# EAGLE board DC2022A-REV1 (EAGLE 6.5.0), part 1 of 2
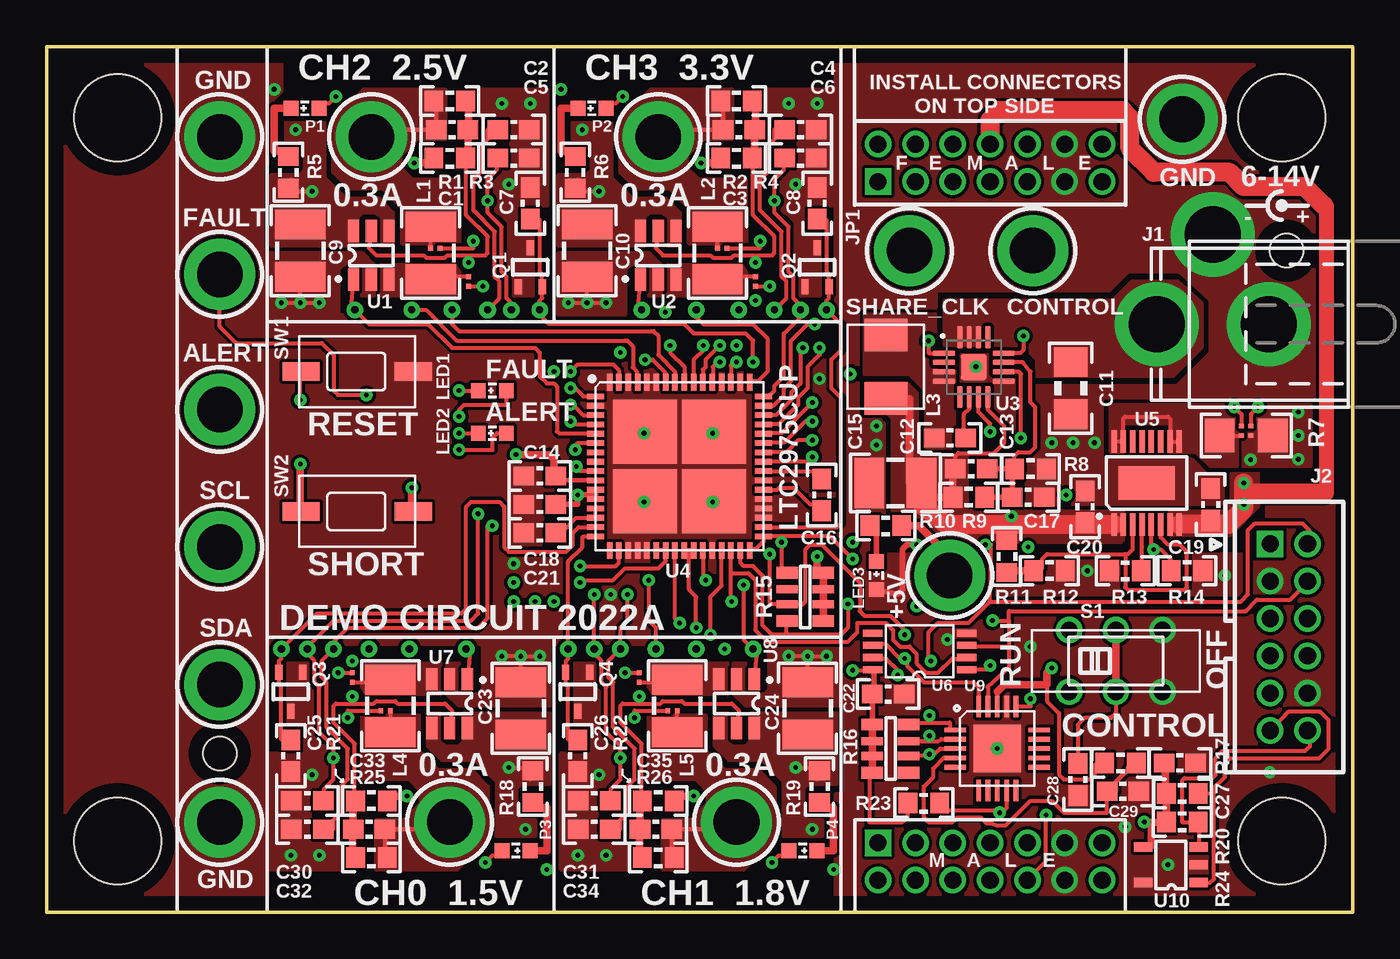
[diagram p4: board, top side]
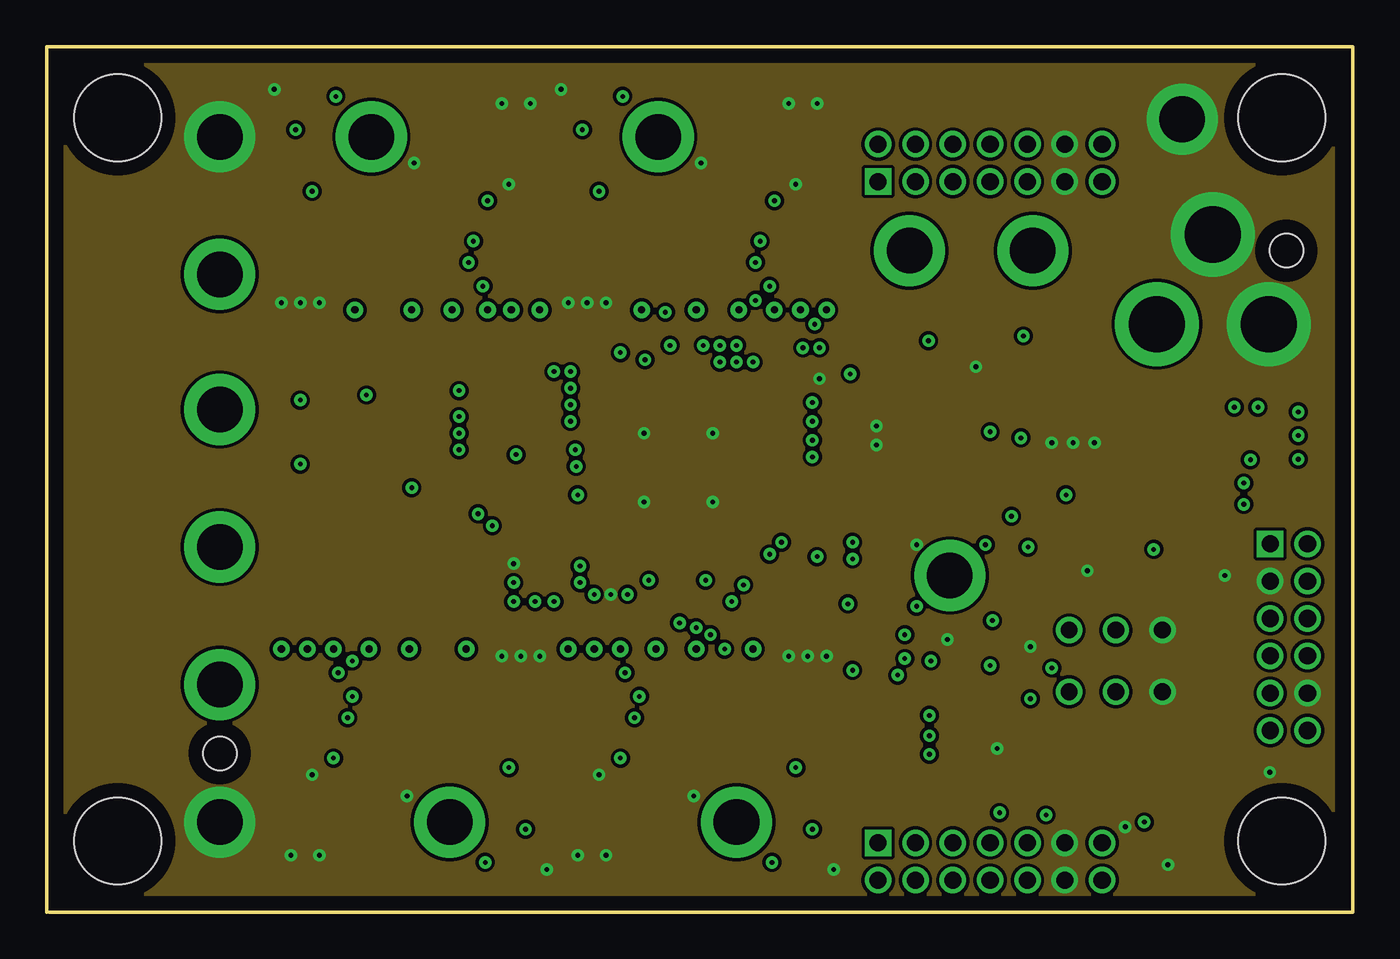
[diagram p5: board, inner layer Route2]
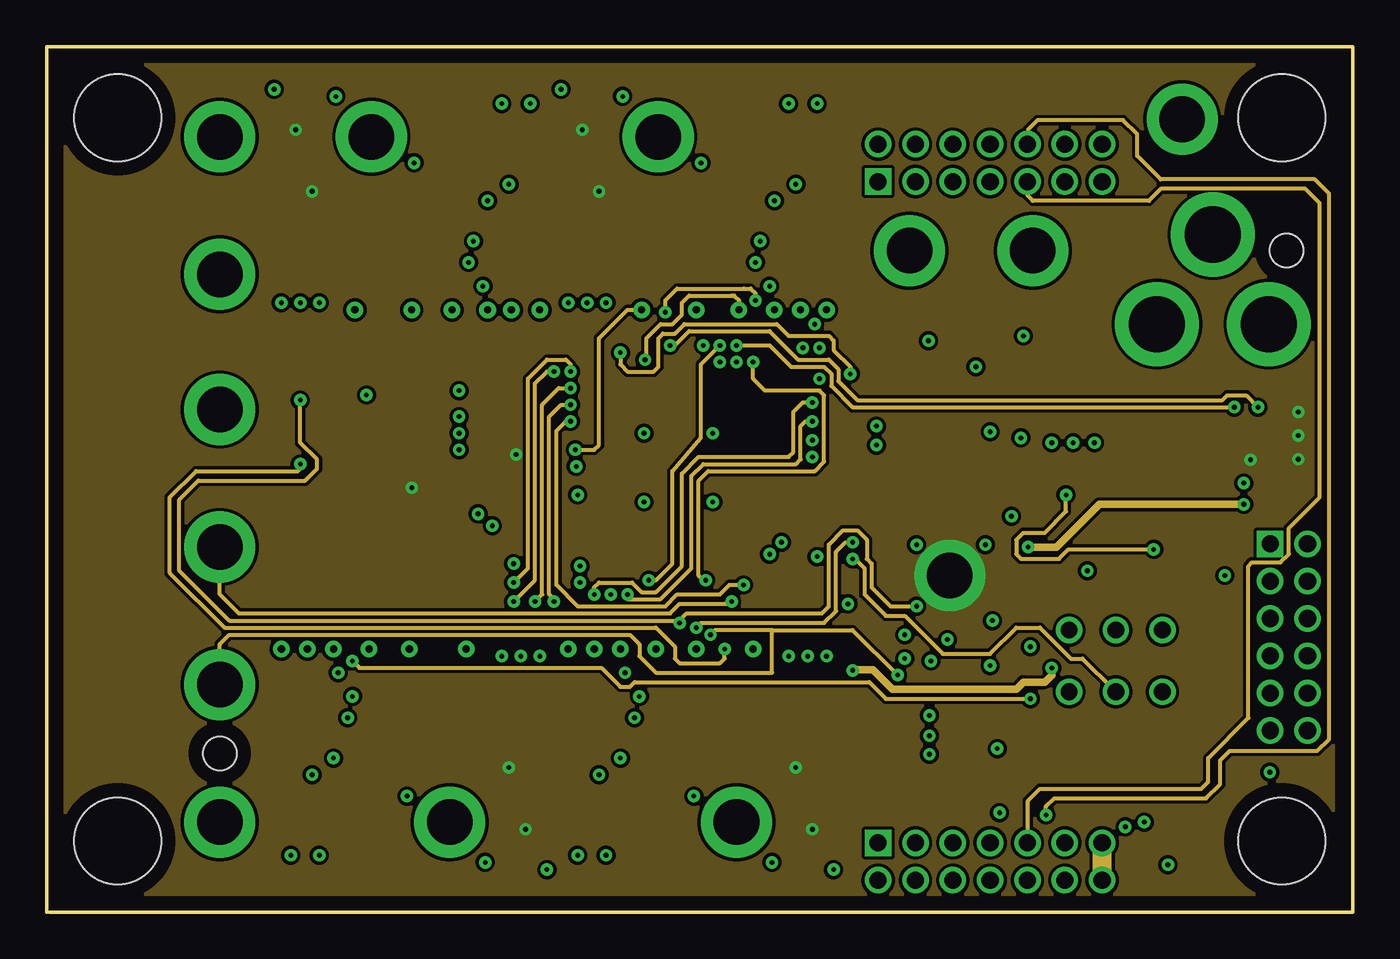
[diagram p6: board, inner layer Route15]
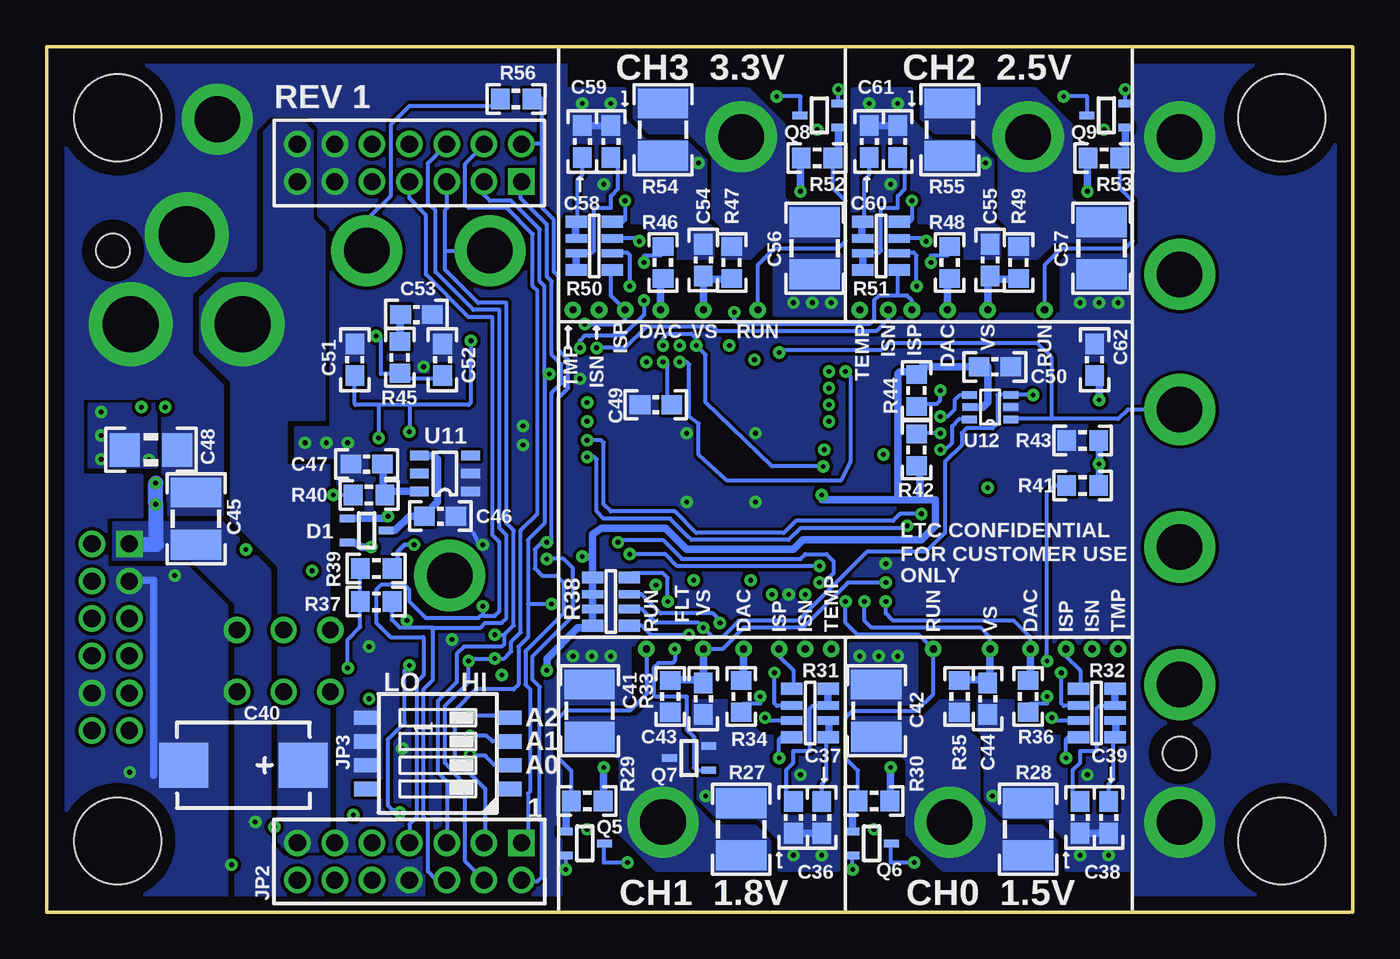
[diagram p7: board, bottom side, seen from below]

Size 69.98 x 46.35 mm. Coordinates in mm from the lower left corner, seen from the top.
Outline: 0,0 0,46.35 69.98,46.35 69.98,0 0.13,0
Copper layers (1*2+15*16): Top 0.035mm / dielectric 1.5mm / Route2 0.035mm / dielectric 0.15mm / Route15 0.035mm / dielectric 0.2mm / Bottom 0.035mm
Design rules "default *": minimum track width 8mil, minimum drill 10mil, track to track 7mil, track to pad 7mil, pad to pad 7mil, via to via 7mil, smd to smd 4mil, copper to edge 30mil, drill to drill 15mil, minimum pad ring 10mil, minimum via ring 8mil, stop-mask expansion 4mil, vias tented up to drill 16mil, thermal gap 10mil
Holes 4.65 mm at 3.81,3.81 3.81,42.55 66.17,42.55 66.17,3.81
Holes 1.8 mm at 66.42,35.43 9.27,8.51

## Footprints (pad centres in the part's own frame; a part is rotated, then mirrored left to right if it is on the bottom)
C0603_BOX = smd 1.1 x 1: 1 -0.85,0; 2 0.85,0
C1210_BOX = smd 1.6 x 2.7: 1 -1.4,0; 2 1.4,0
C1206_BOX = smd 1.6 x 1.8: 1 -1.4,0; 2 1.4,0
C7343 = smd 2.6 x 2.4: + -3.2,0; - 3.2,0
SC70-3 = smd 0.4 x 0.8: 1 -0.65,-1.052; 2 0.65,-1.052; 3 0,1.052
PJ-002A = drill 3 pad 4.5: 1 -3,0; 2 0,-4.8; 3 3,0
CONN_DC1613 = drill 0.914 square: 1 -5,-1 | drill 0.914: 2 -5,1; 3 -3,-1; 4 -3,1; 5 -1,-1; 6 -1,1; 7 1,-1; 8 1,1; 9 3,-1; 10 3,1; 11 5,-1; 12 5,1
2X07M = drill 0.914 square: 1 -6,-1 | drill 0.914: 2 -6,1; 3 -4,-1; 4 -4,1; 5 -2,-1; 6 -2,1; 7 0,-1; 8 0,1; 9 2,-1; 10 2,1; 11 4,-1; 12 4,1; 13 6,-1; 14 6,1
SMT_DIP_4 = smd 1.27 x 0.762: 1 -3.861,1.905; 2 -3.861,0.635; 3 -3.861,-0.635; 4 -3.861,-1.905; 5 3.861,-1.905; 6 3.861,-0.635; 7 3.861,0.635; 8 3.861,1.905
L1210 = smd 1.6 x 2.7: 1 -1.4,0; 2 1.4,0
IHLP_1616AB = smd 1.75 x 2.3: 1 -1.7,0; 2 1.7,0
CHIPLED_0603 = smd 0.8 x 0.8: N 0,0.75; P 0,-0.75
NODE_BREAKER = smd 0.254 x 0.254: 1 -0.254,0; 2 0.254,0
R0603_BOX = smd 1 x 1.1: 1 -0.85,0; 2 0.85,0
R1206_BOX = smd 1.6 x 1.803: 1 -1.422,0; 2 1.422,0
R_VISHAY_CRA06S = smd 1.15 x 0.63: R1_1 -0.975,1.295; R1_2 0.975,1.295; R4_1 -0.975,-1.295; R4_2 0.975,-1.295 | smd 1.15 x 0.44: R2_1 -0.975,0.4; R2_2 0.975,0.4; R3_1 -0.975,-0.4; R3_2 0.975,-0.4
R1210_BOX = smd 1.6 x 2.7: 1 -1.4,0; 2 1.4,0
JS202011CQN = drill 0.9: 1 -2.5,1.65; 2 0,1.65; 3 2.5,1.65; 4 -2.5,-1.65; 5 0,-1.65; 6 2.5,-1.65
SWITCH_PTS635 = smd 2 x 1: SW1 -3,0; SW2 3,0
TP1 = drill 2.438 pad 3.81: TP 0,0
VIA = drill 0.381: 1 0,0
SOT-23-6 = smd 1.2 x 0.6: 1 -1.3,0.95; 2 -1.3,0; 3 -1.3,-0.95; 4 1.3,-0.95; 5 1.3,0; 6 1.3,0.95
QFN16_3X3 = smd 1.2 x 0.3: 1 -1.711,0.734; 2 -1.711,0.234; 3 -1.711,-0.266; 4 -1.711,-0.766; 9 1.489,-0.766; 10 1.489,-0.266; 11 1.489,0.234; 12 1.489,0.734 | smd 0.3 x 1.2: 5 -0.861,-1.616; 6 -0.361,-1.616; 7 0.139,-1.616; 8 0.639,-1.616; 13 0.639,1.584; 14 0.139,1.584; 15 -0.361,1.584; 16 -0.861,1.584 | smd 1.4 x 1.4: PAD -0.111,-0.016
QFN64_9X9 = smd 0.9 x 0.3: 1 -4.5,3.75; 2 -4.5,3.25; 3 -4.5,2.75; 4 -4.5,2.25; 5 -4.5,1.75; 6 -4.5,1.25; 7 -4.5,0.75; 8 -4.5,0.25; 9 -4.5,-0.25; 10 -4.5,-0.75; 11 -4.5,-1.25; 12 -4.5,-1.75; 13 -4.5,-2.25; 14 -4.5,-2.75; 15 -4.5,-3.25; 16 -4.5,-3.75; 33 4.5,-3.75; 34 4.5,-3.25; 35 4.5,-2.75; 36 4.5,-2.25; 37 4.5,-1.75; 38 4.5,-1.25; 39 4.5,-0.75; 40 4.5,-0.25; 41 4.5,0.25; 42 4.5,0.75; 43 4.5,1.25; 44 4.5,1.75; 45 4.5,2.25; 46 4.5,2.75; 47 4.5,3.25; 48 4.5,3.75 | smd 0.3 x 0.9: 17 -3.75,-4.5; 18 -3.25,-4.5; 19 -2.75,-4.5; 20 -2.25,-4.5; 21 -1.75,-4.5; 22 -1.25,-4.5; 23 -0.75,-4.5; 24 -0.25,-4.5; 25 0.25,-4.5; 26 0.75,-4.5; 27 1.25,-4.5; 28 1.75,-4.5; 29 2.25,-4.5; 30 2.75,-4.5; 31 3.25,-4.5; 32 3.75,-4.5; 49 3.75,4.5; 50 3.25,4.5; 51 2.75,4.5; 52 2.25,4.5; 53 1.75,4.5; 54 1.25,4.5; 55 0.75,4.5; 56 0.25,4.5; 57 -0.25,4.5; 58 -0.75,4.5; 59 -1.25,4.5; 60 -1.75,4.5; 61 -2.25,4.5; 62 -2.75,4.5; 63 -3.25,4.5; 64 -3.75,4.5 | smd 3.429 x 3.429: PAD1 -1.854,1.854; PAD2 1.854,1.854; PAD3 -1.854,-1.854; PAD4 1.854,-1.854
MSOP16_EXP = smd 1.2 x 0.3: 1 -2.213,1.75; 2 -2.213,1.25; 3 -2.213,0.75; 4 -2.213,0.25; 5 -2.213,-0.25; 6 -2.213,-0.75; 7 -2.213,-1.25; 8 -2.213,-1.75; 9 2.213,-1.75; 10 2.213,-1.25; 11 2.213,-0.75; 12 2.213,-0.25; 13 2.213,0.25; 14 2.213,0.75; 15 2.213,1.25; 16 2.213,1.75 | smd 1.778 x 3.048: EXP 0,0
MSOP-8 = smd 1.041 x 0.381: 1 -2.55,0.975; 2 -2.55,0.325; 3 -2.55,-0.325; 4 -2.55,-0.975; 5 2.479,-0.975; 6 2.479,-0.325; 7 2.479,0.325; 8 2.479,0.975
QFN20 = smd 1.143 x 0.254: 1 -2.25,1; 2 -2.25,0.5; 3 -2.25,0; 4 -2.25,-0.5; 5 -2.25,-1; 11 2.25,-1; 12 2.25,-0.5; 13 2.25,0; 14 2.25,0.5; 15 2.25,1 | smd 0.254 x 1.143: 6 -1,-2.25; 7 -0.5,-2.25; 8 0,-2.25; 9 0.5,-2.25; 10 1,-2.25; 16 1,2.25; 17 0.5,2.25; 18 0,2.25; 19 -0.5,2.25; 20 -1,2.25 | smd 2.54 x 2.54: PAD 0,0
SOT-23-5 = smd 1 x 0.5: 1 -1.649,0.95; 2 -1.649,0; 3 -1.649,-0.95; 4 1.333,-0.95; 5 1.333,0.95
SOT-23-6@1 = smd 1 x 0.5: 1 -1.374,1.087; 2 -1.374,0.127; 3 -1.374,-0.833; 4 1.374,-0.833; 5 1.374,0.127; 6 1.374,1.087
SC70-6 = smd 0.4 x 0.8: 1 -0.65,-1.102; 2 0,-1.102; 3 0.65,-1.102; 4 0.65,1.102; 5 0,1.098; 6 -0.65,1.102

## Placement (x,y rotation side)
$$U$1  [LT_LOGO_LARGE_SM]  5.46,6.1 90 top
$$U$2  [LT_LOGO_LARGE_SM]  2.03,6.1 90 bottom
C1  220p  [C0603_BOX]  21.72,41.91 0 top
C2  2.2n  [C0603_BOX]  25.02,41.91 0 top
C3  220p  [C0603_BOX]  37.08,41.91 0 top
C4  2.2n  [C0603_BOX]  40.39,41.91 0 top
C5  2.2n  [C0603_BOX]  25.02,40.39 0 top
C6  2.2n  [C0603_BOX]  40.39,40.39 0 top
C7  100n  [C0603_BOX]  25.91,37.97 90 top
C8  100n  [C0603_BOX]  41.27,37.97 90 top
C9  22u/10V  [C1210_BOX]  13.59,35.43 270 top
C10  22u/10V  [C1210_BOX]  28.96,35.43 270 top
C11  10u/25V  [C1206_BOX]  54.86,28.07 90 top
C12  100n  [C0603_BOX]  48.39,25.4 0 top
C13  68p  [C0603_BOX]  49.53,23.75 0 top
C14  1u  [C0603_BOX]  26.42,23.37 0 top
C15  22u/10V  [C1210_BOX]  45.47,22.99 180 top
C16  100n  [C0603_BOX]  41.53,22.35 270 top
C17  47p  [C0603_BOX]  52.58,22.23 0 top
C18  100n  [C0603_BOX]  26.42,21.84 0 top
C19  1u  [C0603_BOX]  62.36,21.84 90 top
C20  1u  [C0603_BOX]  55.63,21.72 90 top
C21  100n  [C0603_BOX]  26.42,20.32 0 top
C22  100n  [C0603_BOX]  45.09,11.68 0 top
C23  22u/10V  [C1210_BOX]  25.4,10.92 90 top
C24  22u/10V  [C1210_BOX]  40.77,10.92 90 top
C25  100n  [C0603_BOX]  13.08,8.38 270 top
C26  100n  [C0603_BOX]  28.45,8.38 270 top
C27  1u  [C0603_BOX]  60.71,8 0 top
C28  1u  [C0603_BOX]  55.24,7.11 270 top
C29  1u  [C0603_BOX]  57.66,6.48 0 top
C30  2.2n  [C0603_BOX]  13.97,5.97 180 top
C31  2.2n  [C0603_BOX]  29.34,5.97 180 top
C32  2.2n  [C0603_BOX]  13.97,4.45 180 top
C33  220p  [C0603_BOX]  17.27,4.45 180 top
C34  2.2n  [C0603_BOX]  29.34,4.45 180 top
C35  220p  [C0603_BOX]  32.64,4.45 180 top
C36  10n  [C0603_BOX]  29.97,5.08 90 bottom
C37  10n  [C0603_BOX]  28.45,5.08 270 bottom
C38  10n  [C0603_BOX]  14.61,5.08 90 bottom
C39  10n  [C0603_BOX]  13.08,5.08 270 bottom
C40  47u/16V  [C7343]  59.44,7.87 180 bottom
C41  22u/10V  [C1210_BOX]  40.89,10.79 90 bottom
C42  22u/10V  [C1210_BOX]  25.53,10.79 90 bottom
C43  100n  [C0603_BOX]  34.8,11.43 90 bottom
C44  100n  [C0603_BOX]  19.56,11.43 90 bottom
C45  22u/10V  [C1210_BOX]  61.98,21.08 90 bottom
C46  1u  [C0603_BOX]  48.9,21.21 0 bottom
C47  4.7u  [C0603_BOX]  52.83,24 0 bottom
C48  10u/25V  [C1206_BOX]  64.39,24.77 0 bottom
C49  10n  [C0603_BOX]  37.34,27.18 0 bottom
C50  100n  [C0603_BOX]  19.18,29.21 0 bottom
C51  4.7u  [C0603_BOX]  53.47,29.59 90 bottom
C52  4.7p  [C0603_BOX]  48.77,29.59 90 bottom
C53  68p  [C0603_BOX]  50.16,32 0 bottom
C54  100n  [C0603_BOX]  34.8,34.92 270 bottom
C55  100n  [C0603_BOX]  19.43,34.92 270 bottom
C56  22u/10V  [C1210_BOX]  28.83,35.56 270 bottom
C57  22u/10V  [C1210_BOX]  13.46,35.56 270 bottom
C58  10n  [C0603_BOX]  41.27,41.27 90 bottom
C59  10n  [C0603_BOX]  39.75,41.27 270 bottom
C60  10n  [C0603_BOX]  25.91,41.27 90 bottom
C61  10n  [C0603_BOX]  24.38,41.27 270 bottom
C62  10n  [C0603_BOX]  13.84,29.59 270 bottom
D1  BAT30CWFILM  [SC70-3]  52.83,20.45 270 bottom
DRILEGEND  [DRILEGEND]  not placed on the board
J1  PJ-002A  [PJ-002A]  62.48,31.5 180 top
J2  CONN_DC1613  [CONN_DC1613]  66.55,14.73 270 top
JP1  FEMALE  [2X07M]  50.55,40.13 0 top
JP2  MALE  [2X07M]  50.55,2.72 180 bottom
JP3  TDA04H0SK1  [SMT_DIP_4]  49.02,8.51 0 bottom
L1  4.7uH  [L1210]  20.57,35.31 90 top
L2  4.7uH  [L1210]  35.94,35.31 90 top
L3  2.2uH  [IHLP_1616AB]  44.96,29.21 270 top
L4  4.7uH  [L1210]  18.41,11.05 270 top
L5  4.7uH  [L1210]  33.78,11.05 270 top
LED1  RED  [CHIPLED_0603]  23.88,27.94 270 top
LED2  RED  [CHIPLED_0603]  23.88,25.65 270 top
LED3  GREEN  [CHIPLED_0603]  44.45,18.03 180 top
NB1  NODE_BREAKER  [NODE_BREAKER]  20.83,35.56 180 top
NB2  NODE_BREAKER  [NODE_BREAKER]  36.2,35.56 180 top
NB3  NODE_BREAKER  [NODE_BREAKER]  22.61,33.78 90 top
NB4  NODE_BREAKER  [NODE_BREAKER]  37.97,33.78 90 top
NB5  NODE_BREAKER  [NODE_BREAKER]  64.01,25.78 90 top
NB6  NODE_BREAKER  [NODE_BREAKER]  64.52,25.78 90 top
NB7  NODE_BREAKER  [NODE_BREAKER]  16.38,12.57 270 top
NB8  NODE_BREAKER  [NODE_BREAKER]  31.75,12.57 270 top
NB9  NODE_BREAKER  [NODE_BREAKER]  18.16,10.79 0 top
NB10  NODE_BREAKER  [NODE_BREAKER]  33.53,10.79 0 top
P1  GREEN  [CHIPLED_0603]  13.84,43.05 270 top
P2  GREEN  [CHIPLED_0603]  29.21,43.05 270 top
P3  GREEN  [CHIPLED_0603]  25.15,3.3 90 top
P4  GREEN  [CHIPLED_0603]  40.51,3.3 90 top
Q1  MMBT3906  [SC70-3]  25.91,34.54 0 top
Q2  MMBT3906  [SC70-3]  41.27,34.54 0 top
Q3  MMBT3906  [SC70-3]  13.08,11.81 180 top
Q4  MMBT3906  [SC70-3]  28.45,11.81 180 top
Q5  DMG1012UW-7  [SC70-3]  41.15,3.68 270 bottom
Q6  DMG1012UW-7  [SC70-3]  25.78,3.68 270 bottom
Q7  DMG1012UW-7  [SC70-3]  35.56,8.26 90 bottom
Q8  DMG1012UW-7  [SC70-3]  28.57,42.67 90 bottom
Q9  DMG1012UW-7  [SC70-3]  13.21,42.67 90 bottom
Q10  SI1304  [SC70-3]  not placed on the board
R1  100k  [R0603_BOX]  21.59,43.43 180 top
R2  100k  [R0603_BOX]  36.96,43.43 180 top
R3  47.5k  [R0603_BOX]  21.59,40.39 0 top
R4  32.4k  [R0603_BOX]  36.96,40.39 0 top
R5  3.01k  [R0603_BOX]  12.95,39.62 270 top
R6  3.01k  [R0603_BOX]  28.32,39.62 270 top
R7  0.050  [R1206_BOX]  64.26,25.53 0 top
R8  10k  [R0603_BOX]  52.7,23.75 180 top
R9  73.2k  [R0603_BOX]  49.4,22.23 180 top
R10  3.01k  [R0603_BOX]  44.96,20.7 0 top
R11  46.4k  [R0603_BOX]  51.44,19.05 90 top
R12  10k  [R0603_BOX]  53.72,18.29 180 top
R13  249  [R0603_BOX]  57.78,18.29 0 top
R14  1.0k  [R0603_BOX]  61.09,18.29 180 top
R15  10k, 4X  [R_VISHAY_CRA06S]  40.64,16.89 0 top
R16  10k, 4X  [R_VISHAY_CRA06S]  45.21,8.76 180 top
R17  249  [R0603_BOX]  57.53,8 0 top
R18  3.01k  [R0603_BOX]  26.04,6.73 90 top
R19  3.01k  [R0603_BOX]  41.4,6.73 90 top
R20  10k  [R0603_BOX]  60.83,6.35 180 top
R21  115k  [R0603_BOX]  17.4,5.97 180 top
R22  80.6k  [R0603_BOX]  32.77,5.97 180 top
R23  10k  [R0603_BOX]  46.99,5.84 0 top
R24  10k  [R0603_BOX]  60.83,4.83 180 top
R25  100k  [R0603_BOX]  17.4,2.92 0 top
R26  100k  [R0603_BOX]  32.77,2.92 0 top
R27  330  [R1210_BOX]  32.77,4.45 270 bottom
R28  330  [R1210_BOX]  17.4,4.45 270 bottom
R29  100k  [R0603_BOX]  41.02,5.97 0 bottom
R30  100k  [R0603_BOX]  25.65,5.97 0 bottom
R31  2.7k, 4X  [R_VISHAY_CRA06S]  29.08,10.67 0 bottom
R32  2.7k, 4X  [R_VISHAY_CRA06S]  13.72,10.67 0 bottom
R33  100  [R0603_BOX]  36.58,11.56 90 bottom
R34  340k  [R0603_BOX]  32.77,11.56 90 bottom
R35  100  [R0603_BOX]  21.08,11.56 90 bottom
R36  402k  [R0603_BOX]  17.4,11.56 90 bottom
R37  10k  [R0603_BOX]  52.32,16.64 0 bottom
R38  10k, 4X  [R_VISHAY_CRA06S]  39.75,16.64 180 bottom
R39  10k  [R0603_BOX]  52.32,18.41 0 bottom
R40  2.49k  [R0603_BOX]  52.7,22.35 0 bottom
R41  OPT  [R0603_BOX]  14.48,22.86 0 bottom
R42  698  [R0603_BOX]  23.37,24.77 270 bottom
R43  100k  [R0603_BOX]  14.48,25.27 0 bottom
R44  698  [R0603_BOX]  23.37,27.94 270 bottom
R45  73.2k  [R0603_BOX]  51.05,29.72 270 bottom
R46  158k  [R0603_BOX]  36.96,34.8 270 bottom
R47  100  [R0603_BOX]  33.27,34.8 270 bottom
R48  210k  [R0603_BOX]  21.59,34.8 270 bottom
R49  100  [R0603_BOX]  17.91,34.8 270 bottom
R50  2.7k, 4X  [R_VISHAY_CRA06S]  40.64,35.69 180 bottom
R51  2.7k, 4X  [R_VISHAY_CRA06S]  25.27,35.69 180 bottom
R52  100k  [R0603_BOX]  28.7,40.39 180 bottom
R53  100k  [R0603_BOX]  13.34,40.39 180 bottom
R54  330  [R1210_BOX]  36.96,41.91 90 bottom
R55  330  [R1210_BOX]  21.59,41.91 90 bottom
R56  10k  [R0603_BOX]  44.83,43.56 0 bottom
S1  CONTROL  [JS202011CQN]  57.28,13.46 0 top
SW1  PTS635SL25SMTR LFS  [SWITCH_PTS635]  16.64,28.96 0 top
SW2  PTS635SK25SMTR LFS  [SWITCH_PTS635]  16.64,21.46 0 top
TP1  TESTPOINT_BIG  [TP1]  60.83,42.47 0 top
TP2  TESTPOINT_BIG  [TP1]  9.27,41.53 0 top
TP3  TESTPOINT_BIG  [TP1]  17.4,41.53 90 top
TP4  TESTPOINT_BIG  [TP1]  32.77,41.53 90 top
TP5  TESTPOINT_BIG  [TP1]  46.23,35.43 0 top
TP6  TESTPOINT_BIG  [TP1]  52.83,35.43 0 top
TP7  TESTPOINT_BIG  [TP1]  9.27,34.16 0 top
TP8  TESPOINT_SMD  [VIA]  16.51,32.26 180 top
TP9  TESPOINT_SMD  [VIA]  26.42,32.26 0 top
TP10  TESPOINT_SMD  [VIA]  31.88,32.26 180 top
TP11  TESPOINT_SMD  [VIA]  41.78,32.26 0 top
TP12  TESTPOINT_BIG  [TP1]  9.27,26.92 0 top
TP13  TESTPOINT_BIG  [TP1]  9.27,19.56 0 top
TP14  TESTPOINT_BIG  [TP1]  48.39,18.03 0 top
TP15  TESPOINT_SMD  [VIA]  12.57,14.1 180 top
TP16  TESPOINT_SMD  [VIA]  22.48,14.1 0 top
TP17  TESPOINT_SMD  [VIA]  27.94,14.1 180 top
TP18  TESPOINT_SMD  [VIA]  37.85,14.1 0 top
TP19  TESTPOINT_BIG  [TP1]  9.27,12.19 0 top
TP20  TESTPOINT_BIG  [TP1]  9.27,4.83 0 top
TP21  TESTPOINT_BIG  [TP1]  21.59,4.83 270 top
TP22  TESTPOINT_BIG  [TP1]  36.96,4.83 270 top
TP23  TESPOINT_SMD  [VIA]  34.8,14.1 0 bottom
TP24  TESPOINT_SMD  [VIA]  32.64,14.1 0 bottom
TP25  TESPOINT_SMD  [VIA]  30.73,14.1 180 bottom
TP26  TESPOINT_SMD  [VIA]  29.34,14.1 180 bottom
TP27  TESPOINT_SMD  [VIA]  19.43,14.1 0 bottom
TP28  TESPOINT_SMD  [VIA]  17.27,14.1 0 bottom
TP29  TESPOINT_SMD  [VIA]  15.37,14.1 180 bottom
TP30  TESPOINT_SMD  [VIA]  13.97,14.1 180 bottom
TP31  TESPOINT_SMD  [VIA]  40.39,32.26 0 bottom
TP32  TESPOINT_SMD  [VIA]  38.99,32.26 0 bottom
TP33  TESPOINT_SMD  [VIA]  37.08,32.26 180 bottom
TP34  TESPOINT_SMD  [VIA]  34.8,32.26 180 bottom
TP35  TESPOINT_SMD  [VIA]  24.89,32.26 0 bottom
TP36  TESPOINT_SMD  [VIA]  23.62,32.26 0 bottom
TP37  TESPOINT_SMD  [VIA]  21.72,32.26 180 bottom
TP38  TESPOINT_SMD  [VIA]  19.56,32.26 180 bottom
U1  LTC3405AES6  [SOT-23-6]  17.4,35.18 90 top
U2  LTC3405AES6  [SOT-23-6]  32.77,35.18 90 top
U3  LTC3604IUD  [QFN16_3X3]  49.78,29.21 0 top
U4  LTC2975CUP  [QFN64_9X9]  33.91,23.88 0 top
U5  LTC4415IMSE  [MSOP16_EXP]  58.93,22.99 90 top
U6  LTC4313CMS8  [MSOP-8]  46.74,13.97 180 top
U7  LTC3405AES6  [SOT-23-6]  21.59,11.18 270 top
U8  LTC3405AES6  [SOT-23-6]  36.96,11.18 270 top
U9  MCP23008-E/ML  [QFN20]  50.93,8.76 0 top
U10  24AA02T-I/OT  [SOT-23-5]  60.07,2.54 180 top
U11  LT6654BMPS6-1.25  [SOT-23-6@1]  48.64,23.62 180 bottom
U12  SN74LVC2G34DCK  [SC70-6]  19.43,27.05 90 bottom
U$6  [DC2022_FRAME]  not placed on the board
